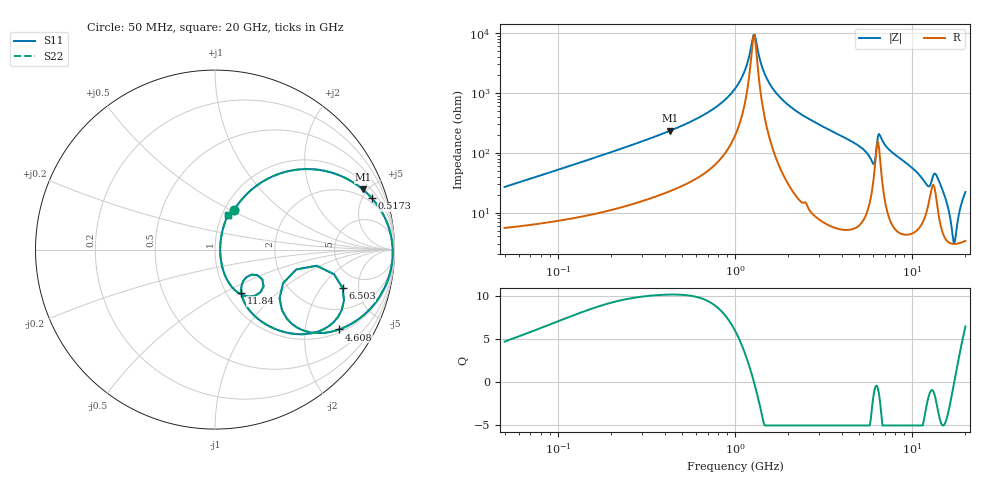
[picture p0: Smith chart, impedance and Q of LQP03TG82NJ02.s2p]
!Murata Part Number: LQP03TG82NJ02
!These Parameters are Measured in Series Mode Connection
!  o--[Z]--o
!Port1  Port2
!  o-------o
!Freq. Start=50[MHz] Stop=20[GHz], 401[Steps]
# Hz S RI R 50
!Freq.(Hz) S11(Real) S11(Imag) S21(Real) S21(Imag) S12(Real) S12(Imag) S22(Real) S22(Imag)
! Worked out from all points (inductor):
!   401 points, 50 MHz to 20 GHz, reference 50 ohm
!   read as one part in series: L = 82.7 nH near 51.52 MHz
!   highest Q = 10.2 at 432.2 MHz (marker M1), where L = 86.2 nH
!   self-resonance near 1.271 GHz
!   S11 on the Smith chart (normalised r, x): 50 MHz: 1.11, +0.52; 517.3 MHz: 1.58, +5.88; 4.608 GHz: 1.11, -3.03; 6.503 GHz: 3.47, -3.31; 11.84 GHz: 1.17, -0.61; 20 GHz: 1.07, +0.44
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5e7  0.1076 0.2219  0.8924 -0.2219  0.8924 -0.2219  0.1076 0.2219
1.364002e8  0.3475 0.4188  0.6525 -0.4188  0.6525 -0.4188  0.3475 0.4188
3.721004e8  0.7742 0.3717  0.2258 -0.3717  0.2258 -0.3717  0.7742 0.3717
4.322267e8  0.8241 0.3349  0.1759 -0.3349  0.1759 -0.3349  0.8241 0.3349
5.173368e8  0.8748 0.2854  0.1252 -0.2854  0.1252 -0.2854  0.8748 0.2854
1e9  0.9796 0.081  0.0204 -0.081  0.0204 -0.081  0.9796 0.081
1.127304e9  0.9864 0.0421  0.0136 -0.0421  0.0136 -0.0421  0.9864 0.0421
1.289994e9  0.9899 -0.00228  0.0101 0.00228  0.0101 0.00228  0.9899 -0.00228
1.454215e9  0.9892 -0.0423  0.0108 0.0423  0.0108 0.0423  0.9892 -0.0423
1.639343e9  0.9848 -0.0831  0.0152 0.0831  0.0152 0.0831  0.9848 -0.0831
2.728004e9  0.9152 -0.2649  0.0848 0.2649  0.0848 0.2649  0.9152 -0.2649
4.608136e9  0.6907 -0.4451  0.3093 0.4451  0.3093 0.4451  0.6907 -0.4451
5.515528e9  0.5084 -0.4557  0.4916 0.4557  0.4916 0.4557  0.5084 -0.4557
5.944466e9  0.3734 -0.3383  0.6266 0.3383  0.6266 0.3383  0.3734 -0.3383
6.217679e9  0.4523 -0.1107  0.5477 0.1107  0.5477 0.1107  0.4523 -0.1107
6.503449e9  0.7109 -0.2136  0.2891 0.2136  0.2891 0.2136  0.7109 -0.2136
7.442007e9  0.5516 -0.4631  0.4484 0.4631  0.4484 0.4631  0.5516 -0.4631
1.183995e10  0.1469 -0.2411  0.8531 0.2411  0.8531 0.2411  0.1469 -0.2411
1.417136e10  0.1559 -0.2545  0.8441 0.2545  0.8441 0.2545  0.1559 -0.2545
1.573793e10  0.0494 -0.1267  0.9506 0.1267  0.9506 0.1267  0.0494 -0.1267
1.721783e10  0.029 -0.00562  0.971 0.00562  0.971 0.00562  0.029 -0.00562
2e10  0.0735 0.1951  0.9265 -0.1951  0.9265 -0.1951  0.0735 0.1951
